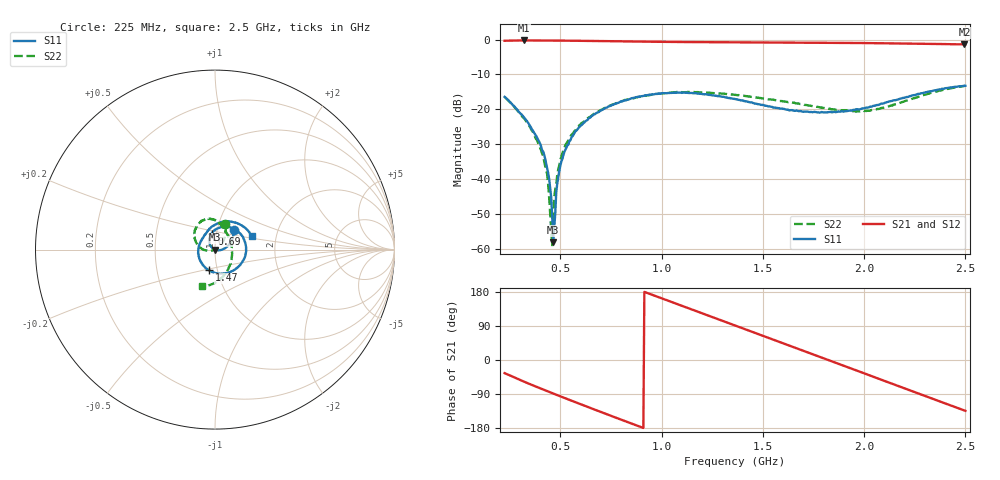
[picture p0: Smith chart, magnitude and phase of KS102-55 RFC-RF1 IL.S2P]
!Agilent	"Technologies,E8364B,MY43040668,A.07.50.67"
!Agilent	E8364B:	A.07.50.67
!Date:	"Tuesday,"	September	"22,"	2015	13:38:02
!Correction:	S11(Full	2	"Port(1,2))"
!S21(Full	2	"Port(1,2))"
!S12(Full	2	"Port(1,2))"
!S22(Full	2	"Port(1,2))"
!S2P	File:	Measurements:	"S11,"	"S21,"	"S12,"	S22:
#	Hz	S	dB	R	50
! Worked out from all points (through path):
!   456 points, 225 MHz to 2.5 GHz, reference 50 ohm
!   highest |S21| = -0.26 dB at 320 MHz (marker M1); lowest = -1.4 dB at 2.495 GHz (marker M2)
!   group delay of S21, straight-line fit = 555 ps
!   lowest |S11| = -58.1 dB at 465 MHz (marker M3), VSWR 1.00, Z = 50.1 - j0.11 ohm
!   |S11| at or under -10 dB: start of sweep to end of sweep
!   |S22| runs from -59.2 to -13.2 dB; largest |S21 - S12| = 0.004
!   S11 on the Smith chart (normalised r, x): 225 MHz: 1.21, +0.27; 690 MHz: 0.95, +0.17; 1.47 GHz: 0.91, -0.21; 2.5 GHz: 1.49, +0.24
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2.25e8  -16.41 45.4  -0.34 -34.6  -0.32 -34.6  -16.37 67.4
3.2e8  -22.25 17.2  -0.26 -57.0  -0.24 -57.0  -22.46 48.8
4.2e8  -32.91 -9.9  -0.27 -78.9  -0.25 -78.8  -34.72 29.4
4.45e8  -39.95 -14.5  -0.28 -84.2  -0.27 -84.2  -45.28 22.3
4.55e8  -45.21 -22.9  -0.29 -86.3  -0.27 -86.3  -54.03 21.1
4.65e8  -58.10 -62.2  -0.29 -88.4  -0.27 -88.5  -53.36 -150.4
4.8e8  -43.70 154.2  -0.29 -91.6  -0.28 -91.6  -41.80 -155.1
4.9e8  -39.40 153.4  -0.30 -93.7  -0.28 -93.7  -37.10 -161.7
5.1e8  -34.24 147.3  -0.31 -97.9  -0.29 -97.9  -32.56 -165.5
6.05e8  -24.50 123.4  -0.36 -117.6  -0.34 -117.6  -23.91 -178.5
6.9e8  -20.77 102.0  -0.42 -135.0  -0.41 -135.0  -20.49 167.8
8.35e8  -17.23 66.3  -0.53 -164.3  -0.52 -164.4  -17.13 145.7
9.85e8  -15.48 29.7  -0.65 165.8  -0.63 165.9  -15.53 125.3
1.19e9  -15.53 -23.4  -0.74 125.3  -0.72 125.4  -15.12 103.1
1.365e9  -17.06 -73.5  -0.80 90.8  -0.78 90.9  -15.83 87.7
1.47e9  -18.42 -105.7  -0.82 70.1  -0.81 70.1  -16.58 79.6
1.745e9  -20.82 170.7  -0.91 15.6  -0.88 15.6  -19.08 53.6
1.93e9  -20.35 129.7  -0.98 -21.2  -0.96 -21.2  -20.43 18.2
2.125e9  -17.70 97.3  -1.08 -60.1  -1.07 -60.0  -19.06 -37.4
2.31e9  -15.04 61.8  -1.23 -96.8  -1.21 -96.7  -15.66 -79.0
2.495e9  -13.26 22.1  -1.40 -133.1  -1.37 -133.1  -13.27 -109.5
2.5e9  -13.24 20.7  -1.38 -134.1  -1.37 -134.1  -13.22 -110.1
